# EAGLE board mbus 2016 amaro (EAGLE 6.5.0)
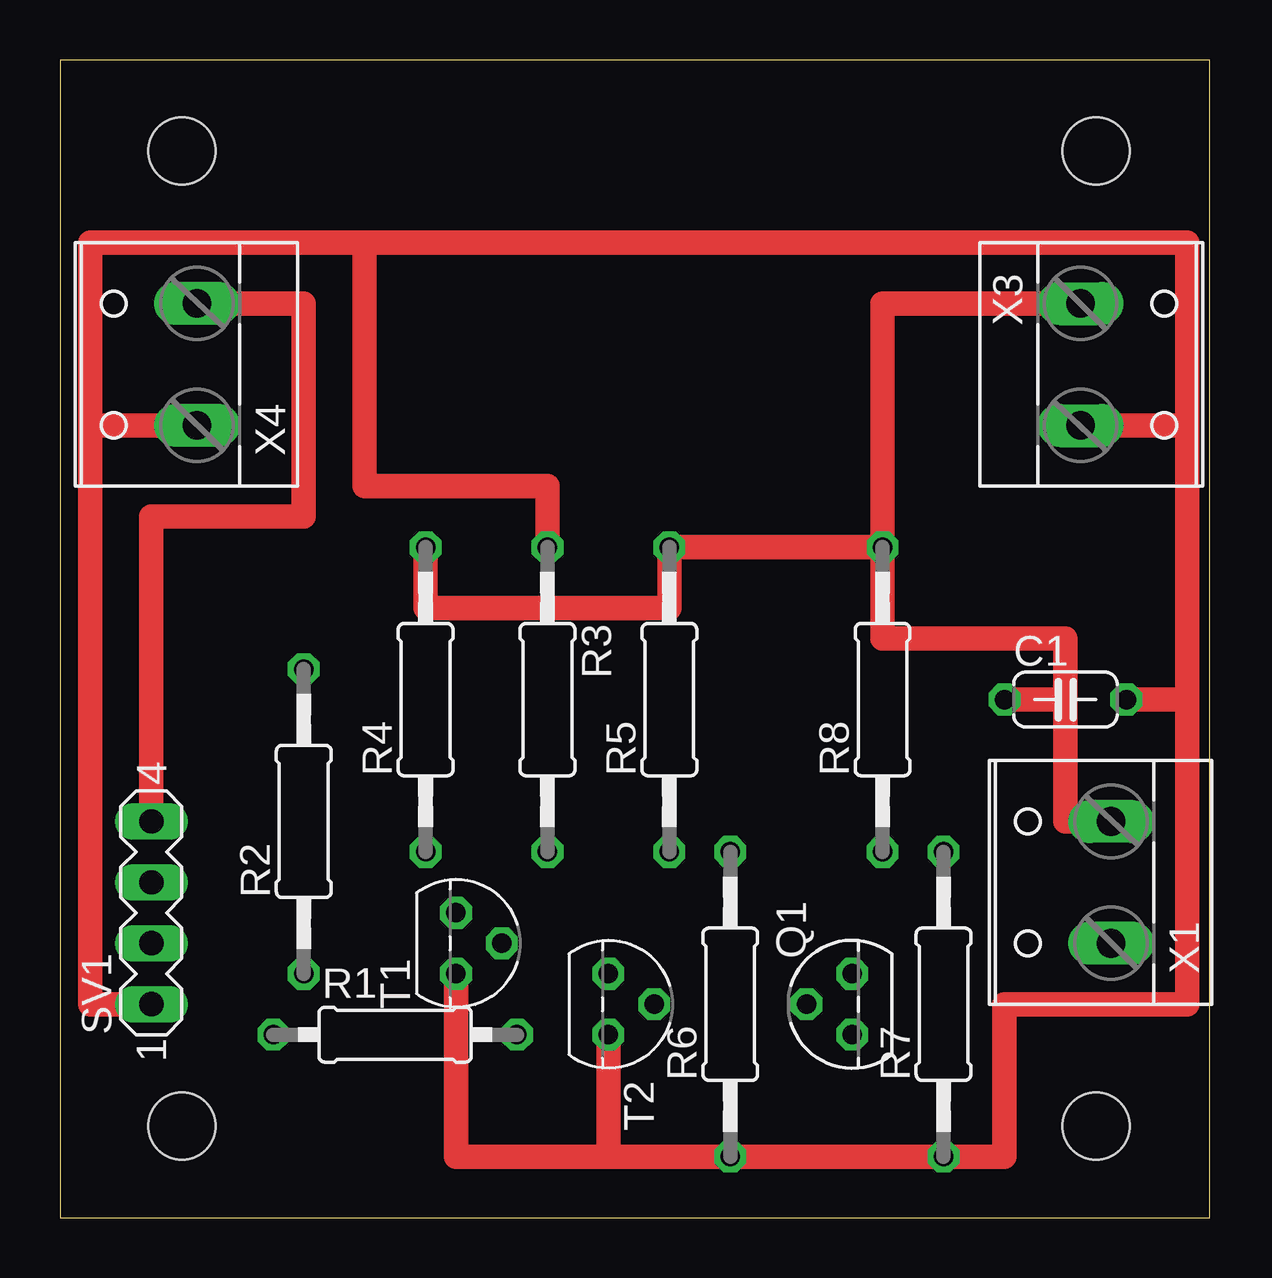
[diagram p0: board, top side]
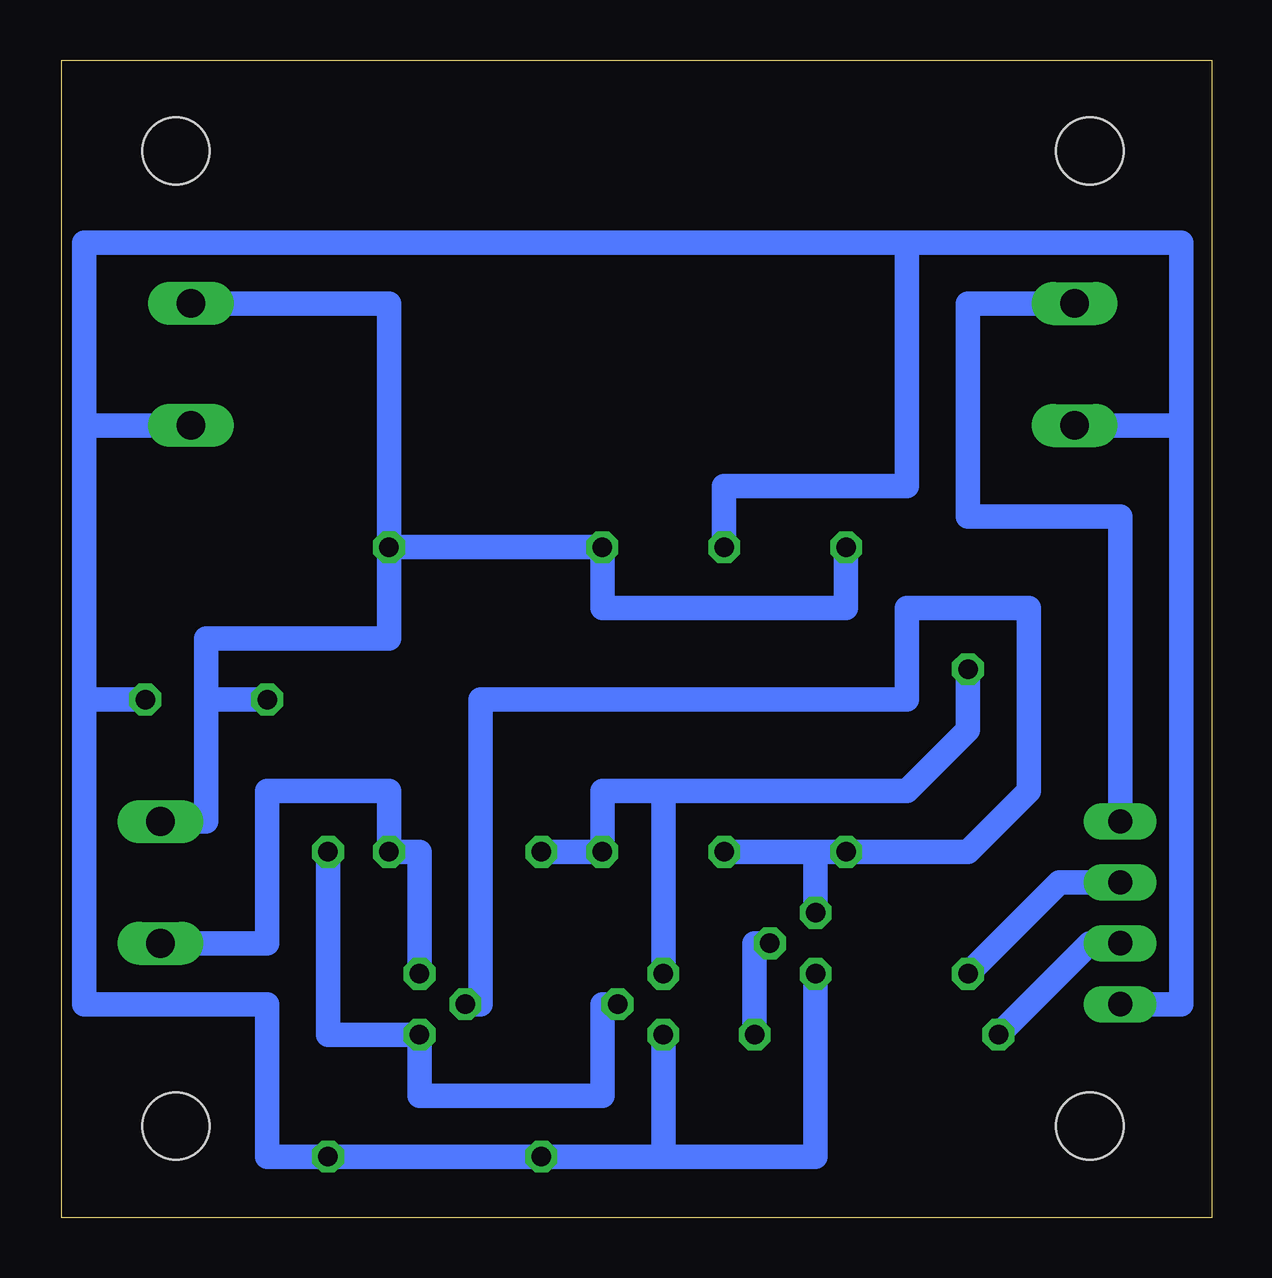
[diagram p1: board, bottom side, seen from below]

Size 47.93 x 48.25 mm. Coordinates in mm from the lower left corner, seen from the top.
Outline: 0,0 47.93,0 47.93,48.25 0,48.25 0,0
Copper layers (1*16): Top 0.035mm / dielectric 1.5mm / Bottom 0.035mm
Design rules "default": minimum track width 10mil, minimum drill 24mil, track to track 8mil, track to pad 8mil, pad to pad 8mil, via to via 8mil, smd to smd 8mil, copper to edge 40mil, drill to drill 8mil, minimum pad ring 10mil, minimum via ring 8mil, stop-mask expansion 4mil, vias tented up to drill 0mil, thermal gap 10mil
Holes 2.8 mm at 43.18,3.81 5.08,44.45 43.18,44.45 5.08,3.81

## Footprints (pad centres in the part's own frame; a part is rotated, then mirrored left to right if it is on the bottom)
C050-024X044 = drill 0.813 octagon: 1 -2.54,0; 2 2.54,0
TO92 = drill 0.813 octagon: 1 1.27,0; 2 0,1.905; 3 -1.27,0
0207/10 = drill 0.813 octagon: 1 -5.08,0; 2 5.08,0
0207/12 = drill 0.813 octagon: 1 -6.35,0; 2 6.35,0
MA04-1 = drill 1.016 long: 1 -3.81,0; 2 -1.27,0; 3 1.27,0; 4 3.81,0
W237-132 = drill 1.194 long: 1 -2.54,-0.635; 2 2.54,-0.635

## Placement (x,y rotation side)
C1  [C050-024X044]  41.91,21.59 0 top
Q1  BC327  [TO92]  33.02,8.89 90 top
R1  1k  [0207/10]  13.97,7.62 0 top
R2  560R  [0207/12]  10.16,16.51 90 top
R3  22k  [0207/12]  20.32,21.59 270 top
R4  33k  [0207/12]  15.24,21.59 90 top
R5  33k  [0207/12]  25.4,21.59 90 top
R6  3k3  [0207/12]  27.94,8.89 90 top
R7  82R  [0207/12]  36.83,8.89 90 top
R8  220k  [0207/12]  34.29,21.59 90 top
SV1  [MA04-1]  3.81,12.7 90 top
T1  BC337  [TO92]  16.51,11.43 270 top
T2  BC337  [TO92]  22.86,8.89 270 top
X1  [W237-132]  43.18,13.97 90 top
X3  [W237-132]  43.18,35.56 270 top
X4  [W237-132]  5.08,35.56 90 top

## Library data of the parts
C1 R1-R8 = resistor
Q1 = transistor-pnp
SV1 = con-lstb; OC_FARNELL: unknown; OC_NEWARK: unknown
T1 T2 = transistor
X1 X3 X4 = con-wago-508; OC_FARNELL: unknown; OC_NEWARK: unknown

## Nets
GND: C1.2 R3.1 R6.1 R7.1 SV1.1 T1.1 T2.1 X3.2 X4.1
N$1: R1.2 T1.2
N$2: R2.2 R5.1 R6.2 T2.3
N$3: Q1.3 R7.2 T2.2
N$4: Q1.1 R8.1 X1.1
N$5: SV1.4 X4.2
N$6: C1.1 R4.2 R5.2 R8.2 X1.2 X3.1
N$7: Q1.2 R3.2 R4.1 T1.3
N$8: R2.1 SV1.3
N$9: R1.1 SV1.2

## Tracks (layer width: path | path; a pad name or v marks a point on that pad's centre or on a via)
GND
  Top 1.016: SV1.1 1.27,8.89 1.27,33.02 | 5.08,33.02 1.27,33.02 | 1.27,33.02 1.27,40.64 12.7,40.64 | 12.7,40.64 46.99,40.64 46.99,33.02 | 46.99,33.02 43.18,33.02 | C1.2 46.99,21.59 | 46.99,21.59 46.99,33.02 | 46.99,21.59 46.99,8.89 39.37,8.89 39.37,2.54 22.86,2.54 | 22.86,2.54 16.51,2.54 T1.1 | R3.1 20.32,30.48 12.7,30.48 12.7,40.64 | 22.86,2.54 T2.1
  Bottom 1.016: 22.86,2.54 R6.1 R7.1 39.37,2.54 39.37,8.89 46.99,8.89 46.99,21.59 | T2.1 22.86,2.54 | T1.1 16.51,2.54 22.86,2.54 | R3.1 20.32,30.48 12.7,30.48 12.7,40.64 | 46.99,21.59 46.99,33.02 | 46.99,33.02 X3.2 | X4.1 1.27,33.02 | 1.27,33.02 1.27,8.89 SV1.1 | 12.7,40.64 1.27,40.64 1.27,33.02 | 46.99,33.02 46.99,40.64 12.7,40.64 | C1.2 46.99,21.59
N$1
  Bottom 1.016: T1.2 19.05,11.43 R1.2
N$2
  Bottom 1.016: R2.2 10.16,20.32 12.7,17.78 22.86,17.78 | 22.86,17.78 25.4,17.78 R5.1 R6.2 | T2.3 22.86,17.78
N$3
  Bottom 1.016: T2.2 25.4,8.89 25.4,5.08 33.02,5.08 Q1.3 36.83,7.62 R7.2
N$4
  Bottom 1.016: Q1.1 33.02,15.24 R8.1 34.29,17.78 39.37,17.78 39.37,11.43 X1.1
N$5
  Top 1.016: SV1.4 3.81,29.21 10.16,29.21 10.16,38.1 6.35,38.1
  Bottom 1.016: X4.2 10.16,38.1 10.16,29.21 3.81,29.21 SV1.4
N$6
  Top 1.016: R4.2 15.24,25.4 25.4,25.4 R5.2 R8.2 | R8.2 34.29,24.13 41.91,24.13 41.91,21.59 | 41.91,21.59 41.91,16.51 44.45,16.51 | C1.1 41.91,21.59 | R8.2 34.29,38.1 43.18,38.1
  Bottom 1.016: R4.2 15.24,25.4 25.4,25.4 R5.2 R8.2 | R8.2 34.29,24.13 41.91,24.13 41.91,21.59 | X1.2 41.91,16.51 41.91,21.59 | X3.1 34.29,38.1 R8.2 | C1.1 41.91,21.59
N$7
  Bottom 1.016: T1.3 16.51,15.24 | Q1.2 30.48,8.89 30.48,21.59 12.7,21.59 12.7,25.4 7.62,25.4 7.62,17.78 10.16,15.24 R4.1 16.51,15.24 | 16.51,15.24 R3.2
N$8
  Bottom 1.016: R2.1 6.35,13.97 SV1.3
N$9
  Bottom 1.016: R1.1 5.08,11.43 SV1.2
